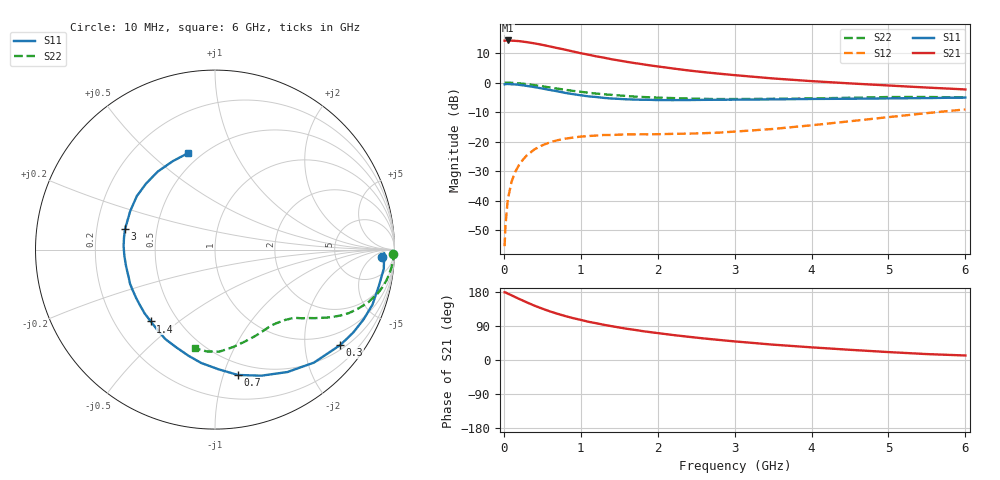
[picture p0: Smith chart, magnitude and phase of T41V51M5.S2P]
! Infineon Technologies  Discrete & RF Semiconductors
! BFR182T
! Si NPN RF Bipolar Junction Transistor in SC75
! VCE = 1.5 V  IC = 1.5 mA
! Common Emitter S-Parameters:  October  1999
# GHz  S  MA  R  50
!  f  S11  S21  S12  S22
! GHz  MAG  ANG  MAG  ANG  MAG  ANG  MAG  ANG
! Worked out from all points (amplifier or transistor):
!   36 points, 10 MHz to 6 GHz, reference 50 ohm
!   highest |S21| = 14.3 dB at 50 MHz (marker M1)
!   |S21| within 3 dB of that: start of sweep to 773.4 MHz
!   unconditionally stable (mu >= 1): 2.118 GHz to 4.539 GHz
!   at 250 MHz: K = 0.12, MSG = 19.9 dB, |S12| = -26.0 dB
!   at 1.4 GHz: K = 0.71, MSG = 12.8 dB, |S12| = -17.7 dB
!   at 6 GHz: K = 0.86, MSG = 3.4 dB, |S12| = -9.1 dB
!   S11 on the Smith chart (normalised r, x): 10 MHz: 21, -13; 300 MHz: 0.62, -2.84; 700 MHz: 0.40, -1.12; 1.4 GHz: 0.36, -0.40; 3 GHz: 0.32, +0.10; 6 GHz: 0.43, +0.67
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0.01  0.9337 -2.4  5.124 178.5  0.0017 81.2  0.9907 -1.3
0.02  0.9429 -1.2  5.122 178.6  0.0036 102.9  0.9916 -1.0
0.05  0.9464 -6.5  5.16 175.2  0.0103 89.6  0.9956 -2.7
0.1  0.9356 -12.3  5.123 170.8  0.0209 83.1  0.9893 -5.3
0.15  0.9293 -19.3  5.085 165.8  0.0312 79.7  0.981 -7.8
0.2  0.9148 -25.1  5.024 161.1  0.0408 76.8  0.9701 -10.3
0.3  0.8774 -37.3  4.826 151.9  0.0588 69.4  0.9404 -14.9
0.4  0.8369 -48.8  4.604 143.2  0.0742 62.7  0.9025 -19.0
0.5  0.7925 -59.4  4.349 135.5  0.0867 58.0  0.8641 -22.3
0.6  0.7485 -69.8  4.083 128.2  0.0976 52.9  0.8254 -25.4
0.7  0.7102 -79.6  3.827 121.8  0.1058 49.5  0.788 -27.8
0.9  0.6362 -97.0  3.354 110.5  0.117 43.4  0.7221 -31.7
1.1  0.5841 -112.3  2.962 100.9  0.1245 39.2  0.6727 -34.6
1.4  0.5368 -131.8  2.48 89.3  0.1296 35.4  0.6187 -38.2
1.6  0.5199 -143.9  2.239 82.4  0.1324 34.5  0.5908 -40.1
1.8  0.5113 -154.0  2.047 76.3  0.1333 34.6  0.5693 -42.5
2.2  0.5041 -169.6  1.73 65.9  0.1354 36.3  0.5457 -46.9
3  0.5141 167.3  1.335 49.1  0.1478 44.4  0.5258 -57.1
3.5  0.5188 155.6  1.173 40.5  0.1639 50.2  0.5306 -64.5
4.5  0.5319 136.2  0.968 26.9  0.2213 56.5  0.5524 -79.6
5.5  0.546 115.5  0.823 15.6  0.3041 55.7  0.5693 -94.5
6  0.5582 105.6  0.765 11.9  0.3512 52.8  0.5615 -101.4
